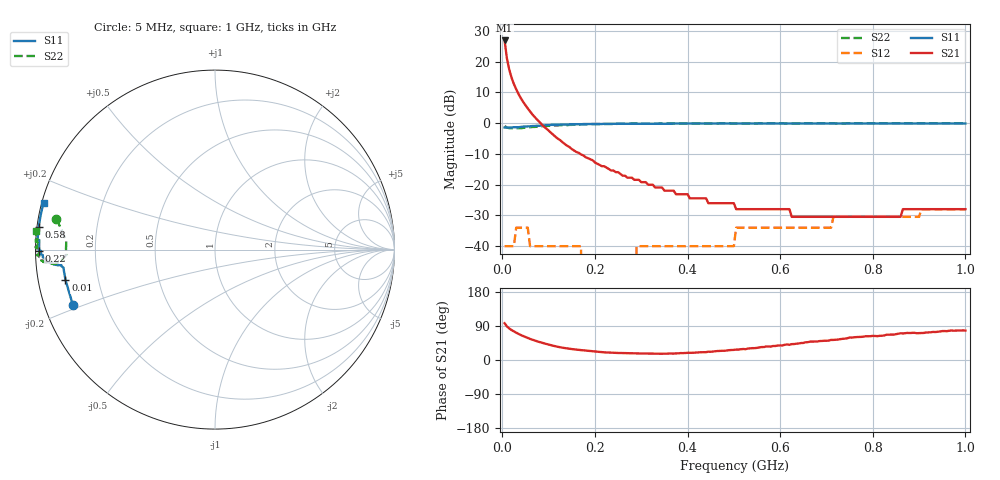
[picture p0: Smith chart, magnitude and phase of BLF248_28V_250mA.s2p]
! Filename:  BLF248_28V_250mA.s2p
! Philips part #: BLF248  !date: 22-05-2003
!Vdd=28V ; Idq=250mA
!D:\Vee measurements\measurement data\VDMOST\BLF248\28V_250mA_#1
# HZ S MA R 50
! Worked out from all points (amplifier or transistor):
!   200 points, 5 MHz to 1 GHz, reference 50 ohm
!   highest |S21| = 26.9 dB at 5 MHz (marker M1)
!   |S21| within 3 dB of that: start of sweep to 7.549 MHz
!   S11 on the Smith chart (normalised r, x): 5 MHz: 0.08, -0.19; 10 MHz: 0.08, -0.10; 220 MHz: 0.01, -0.00; 580 MHz: 0.01, +0.06; 1 GHz: 0.01, +0.13
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5000000  0.85 -158.7  22.19 97.0  0.01 -1.4  0.9 168.9
1e7  0.85 -168.6  11.27 88.5  0.01 20.7  0.85 174.2
1.5e7  0.85 -171.9  7.47 83.2  0.01 21.9  0.83 176.6
2e7  0.85 -173.2  5.51 79.0  0.01 18.2  0.83 178.2
2.5e7  0.86 -173.8  4.35 75.5  0.01 13.4  0.83 179.5
3e7  0.86 -174.1  3.57 72.0  0.02 8.2  0.83 -179.8
4.5e7  0.88 -174.3  2.22 63.2  0.02 -3.8  0.84 -177.2
5.5e7  0.89 -174.5  1.74 58.1  0.02 -10.2  0.85 -176.1
6.5e7  0.9 -174.7  1.39 53.5  0.01 -15.6  0.87 -175.5
9e7  0.92 -175.5  0.88 44.0  0.01 -24.6  0.9 -174.9
1.7e8  0.96 -178.2  0.31 26.1  0.01 -23.2  0.96 -175.9
1.75e8  0.97 -178.4  0.3 25.5  0 -21.2  0.96 -176.0
2.2e8  0.98 -179.7  0.2 20.2  0 15.1  0.97 -177.2
2.85e8  0.98 178.6  0.12 17.7  0 67.6  0.99 -178.2
2.9e8  0.98 178.4  0.12 17.3  0.01 69.2  0.99 -178.3
3.4e8  0.98 177.3  0.09 16.5  0.01 77.6  0.99 -179.0
5e8  0.99 174.2  0.05 26.7  0.01 88.6  0.99 179.0
5.05e8  0.99 174.1  0.04 27.5  0.02 88.5  0.99 179.0
5.8e8  0.99 172.6  0.04 35.4  0.02 89.8  1 178.1
6.7e8  0.99 171.0  0.03 48.6  0.02 90.7  1 177.2
8.35e8  0.99 167.9  0.03 66.8  0.03 93.2  1 175.7
1e9  0.99 164.7  0.04 77.6  0.04 92.3  1 174.1
